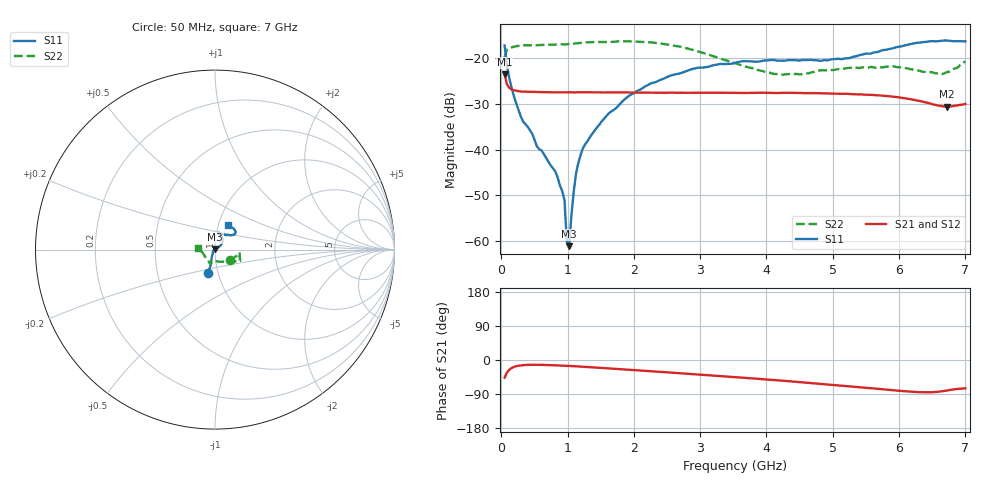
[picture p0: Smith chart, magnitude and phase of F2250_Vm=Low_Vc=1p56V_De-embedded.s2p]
! Integrated Device Technology
! Corporate Headquarters
! 6024 Silver Creek Valley Road
! San Jose, CA 95138  USA
! Phone:  1-408-284-8200
! Toll Free:  1-800-223-1366
! Webpage:  http://www.idt.com/
! Timing and RF Division
! 515 Groton Road, Suite 102
! Westford, MA 01886-6024
! Device:  F2250
! Description: Voltage Variable RF Attenuator
! Frequency:  50.0 -  6000.00 MHz
! Package:  3x3 mm Thin QFN Plastic Package: 16 pin
! Ports:  2 RF, 3 DC
!  Pin  1  = GND
!  Pin  2  = NC
!  Pin  3  = RF1  = Port 1
!  Pin  4  = NC
!  Pin  5  = GND
!  Pin  6  = GND
!  Pin  7  = GND
!  Pin  8  = GND
!  Pin  9  = NC
!  Pin 10  = RF2  = Port 2
!  Pin 11  = NC
!  Pin 12  = GND
!  Pin 13  = GND
!  Pin 14  = VCNTRL
!  Pin 15  = VDD
!  Pin 16  = VMODE
! Vcntrl:  1.560 Volts
! Vmode:  +0.000 Volts
! Vdd:  +3.30  Volts
! Current:  1.188 mA
! Data:  The device was measured on a the F2250 evaluation board which has
!  individual transmission lines to the RF pins.  Data was collected
!  using a calibrated network analyzer.  The evaluation board was
!  de-embedded using a TRL calibration technique.
!  The reference plane is the edge of the package pin.
! Misc:  SN 10
!  Action Tracker AT0258
! Date Measured:  2014-11-26
! Date:  2015-10-15  MJV
! Note:
!  Integrated Device Technology supplies this data as a sample of measured
!  data at the package pin for this product.  Your particular data for this
!  product may vary.
!  Data was taken at 25 degrees C.
!  Integrated Device Technology reserves the right to change this data at anytime.
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# GHz S dB R 50
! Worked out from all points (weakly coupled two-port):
!   201 points, 50 MHz to 7 GHz, reference 50 ohm
!   highest |S21| = -23.47 dB at 50 MHz (marker M1); lowest = -30.6 dB at 6.722 GHz (marker M2)
!   lowest |S11| = -61.2 dB at 1.023 GHz (marker M3), VSWR 1.00, Z = 50 + j0.0794 ohm
!   |S11| at or under -10 dB: start of sweep to end of sweep
!   |S22| runs from -23.6 to -16.3 dB; largest |S21 - S12| = 0.00018
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0.05  -17.18 -107.0  -23.47 -46.6  -23.47 -46.6  -19.77 -36.0
0.1195  -24.29 -108.7  -26.46 -25.8  -26.46 -25.8  -17.77 -11.3
0.29325  -32.70 -120.9  -27.28 -14.3  -27.25 -14.3  -17.17 -8.7
0.5365  -39.28 -145.7  -27.37 -12.6  -27.38 -12.6  -17.12 -10.0
0.8145  -44.77 177.3  -27.46 -14.0  -27.46 -14.0  -16.98 -14.3
0.91875  -49.09 154.6  -27.45 -14.8  -27.44 -14.8  -16.92 -16.2
0.9535  -51.09 178.9  -27.45 -15.1  -27.45 -15.1  -16.98 -16.5
0.98825  -60.24 158.5  -27.45 -15.4  -27.44 -15.4  -16.91 -16.8
1.023  -61.17 65.2  -27.43 -15.7  -27.46 -15.7  -16.86 -16.9
1.05775  -54.40 44.7  -27.44 -16.0  -27.46 -16.0  -16.83 -17.2
1.12725  -45.23 31.4  -27.45 -16.6  -27.46 -16.6  -16.72 -18.4
1.2315  -39.70 28.5  -27.44 -17.7  -27.45 -17.7  -16.57 -20.0
1.5095  -33.91 32.0  -27.47 -20.9  -27.47 -20.9  -16.44 -21.9
1.857  -29.03 35.8  -27.47 -25.0  -27.47 -24.9  -16.28 -24.6
2.37825  -24.86 44.4  -27.53 -31.1  -27.53 -31.1  -16.69 -27.4
2.93425  -22.15 58.0  -27.55 -37.8  -27.54 -37.8  -18.34 -32.7
3.525  -21.00 71.1  -27.57 -45.3  -27.57 -45.3  -21.05 -50.3
4.11575  -20.38 78.8  -27.58 -53.0  -27.60 -52.9  -23.44 -76.8
4.7065  -20.41 71.6  -27.63 -61.3  -27.60 -61.3  -22.99 -101.2
5.85325  -17.95 39.6  -28.32 -78.9  -28.32 -78.9  -21.84 -109.7
6.722  -16.11 49.6  -30.59 -80.3  -30.55 -80.3  -23.01 -163.0
7  -16.27 62.8  -29.99 -74.6  -29.99 -74.6  -20.68 173.8
